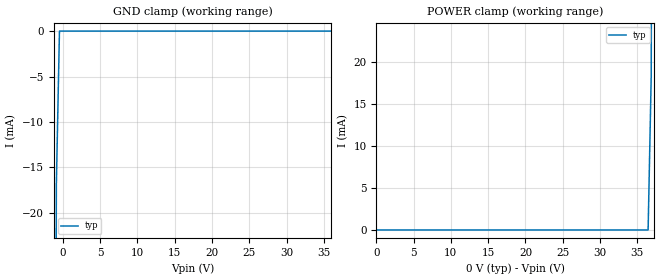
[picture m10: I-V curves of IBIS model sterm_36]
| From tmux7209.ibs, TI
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| sterm_36
[Model]   sterm_36
Model_type   Terminator
|   typ   min   max
C_comp   6.362683e-12   NA   NA
[Voltage Range]   36   0   36
[Temperature Range]   27   NA   NA
[Power Clamp Reference]   0   NA   NA
[GND Clamp Reference]   0   NA   NA
[GND Clamp]
|   Voltage   I(typ)   I(min)   I(max)
-5V       -1.607A    NA         NA
-1.273V   -120.6mA   NA         NA
-858.6mV  -16.83mA   NA         NA
-444.4mV  -1.564uA   NA         NA
36V       883.9pA    NA         NA
[POWER Clamp]
|   Voltage   I(typ)   I(min)   I(max)
0V        -828.1pA   NA         NA
36.44V    1.655uA    NA         NA
36.86V    18.16mA    NA         NA
37.27V    162.9mA    NA         NA
41V       3.304A     NA         NA
